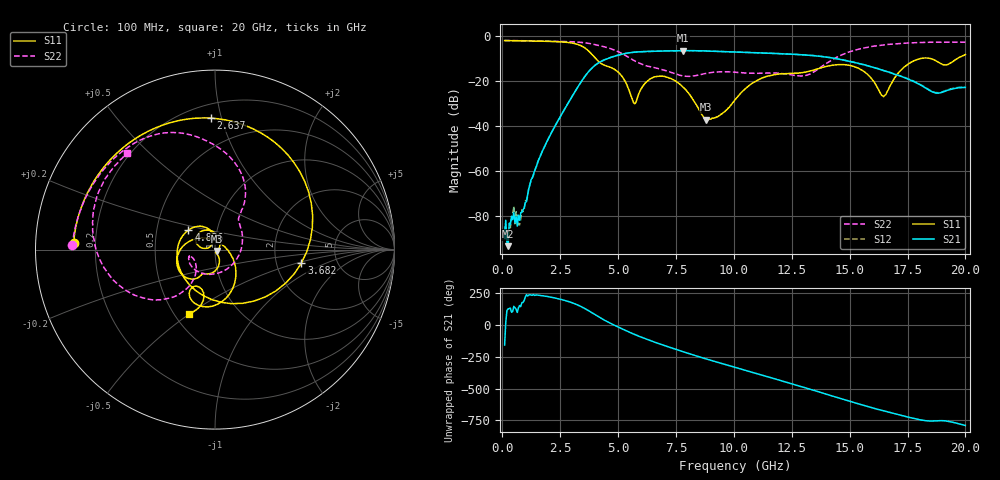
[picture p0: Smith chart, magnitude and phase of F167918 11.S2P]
!  2-Port S-parameters saved by WinCal
! VAR MeasName=S-Parameters (CALIBRATED_DATA) read from VNA (N5242A)
! VAR MeasDate=2016-11-22 10:25:21
! VAR NAME=F167918 11
! VAR FILENAME=F167918 11.S2P
! VAR DATE=2016-11-22 10:25:21
! VAR PHYS_PORTS=1,2
# Hz S DB R 50
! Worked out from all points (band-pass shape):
!   401 points, 100 MHz to 20 GHz, reference 50 ohm
!   highest |S21| = -6.51 dB at 7.811 GHz (marker M1); lowest = -93.3 dB at 249.2 MHz (marker M2)
!   |S21| within 3 dB of the highest: 4.687 GHz to 14.08 GHz (9.396 GHz wide, 100 % of centre)
!   lowest |S11| = -37.2 dB at 8.806 GHz (marker M3), VSWR 1.03, Z = 51.1 - j0.838 ohm
!   |S11| at or under -10 dB: 4.028 GHz to 18.07 GHz (14.04 GHz wide, 127 % of centre); 18.48 GHz to 19.66 GHz (1.178 GHz wide, 6.18 % of centre)
!   |S22| runs from -18.0 to -2.0 dB; largest |S21 - S12| = 0.0034
!   S11 on the Smith chart (normalised r, x): 100 MHz: 0.12, +0.02; 2.637 GHz: 0.29, +0.93; 3.682 GHz: 2.78, -0.55; 4.826 GHz: 0.73, +0.16; 20 GHz: 0.59, -0.50
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1e8  -2.07 177.3  -90.12 -157.8  -84.60 101.3  -2.00 178.3
2.4925e8  -2.08 173.3  -93.35 125.9  -92.31 33.2  -2.02 175.8
8.4625e8  -2.18 157.3  -78.30 175.7  -77.16 -175.3  -2.11 166.4
1.64225e9  -2.32 133.7  -53.39 -127.8  -53.09 -126.9  -2.24 153.6
2.63725e9  -2.70 91.7  -33.45 -163.7  -33.43 -164.2  -2.44 135.3
3.43325e9  -4.51 25.6  -19.93 142.2  -19.95 142.1  -2.88 116.2
3.682e9  -6.25 -8.9  -16.42 117.1  -16.41 117.1  -3.21 109.3
4.32875e9  -12.62 -136.8  -11.00 46.3  -10.95 46.0  -4.62 91.1
4.82625e9  -14.72 143.5  -9.05 -0.8  -9.04 -1.1  -6.21 76.2
5.72175e9  -30.12 138.6  -7.16 -75.0  -7.16 -75.1  -11.12 56.3
6.7665e9  -17.84 138.1  -6.74 -147.2  -6.75 -147.5  -14.57 39.8
7.81125e9  -22.74 75.0  -6.51 149.4  -6.53 149.4  -17.78 -30.6
8.80625e9  -37.21 -36.5  -6.68 92.4  -6.69 92.3  -16.58 -114.1
1.005e10  -28.35 -63.1  -7.11 25.7  -7.12 25.8  -16.12 -159.7
1.189075e10  -16.95 -106.2  -7.84 -70.2  -7.81 -70.1  -16.51 -165.9
1.338325e10  -15.34 -119.2  -8.68 -150.5  -8.64 -150.4  -16.40 -133.7
1.5025e10  -13.12 -164.4  -11.35 118.2  -11.31 118.1  -6.96 -141.4
1.6418e10  -26.54 72.0  -15.24 46.0  -15.16 46.6  -4.01 -171.6
1.67165e10  -22.77 -2.9  -16.12 31.7  -16.15 32.5  -3.71 -177.4
1.786075e10  -10.65 -82.7  -20.68 -19.7  -20.51 -19.2  -2.97 162.8
1.875625e10  -11.20 -121.0  -25.38 -34.6  -25.18 -34.5  -2.77 148.6
2e10  -8.27 -112.0  -22.85 -70.9  -22.64 -71.0  -2.78 132.4
